(* FB_CylinderTempRecord	- number of control signals控制信号的数量:
									one direction is controllable一个方向是可控的
							- type of feedback signal反馈信号的类型:
									feedback in base and work position基准和工作位置的反馈
							- with temperature recording for data analysis具有用于数据分析的温度记录		*)

FUNCTION_BLOCK FB_CylinderTempRecord EXTENDS FB_CylinderTemp
VAR_INPUT
	bRecordStart		: BOOL;								// Signal to start the temperature recording开始温度记录的信号
	tIntervalTime		: TIME;								// Time of intervals to record the temperature记录温度的间隔时间 
END_VAR
VAR_OUTPUT
	bRecordDone			: BOOL;								// True if the temperature recording is done如果完成温度记录，则为True
	aTemps				: ARRAY[1..100] OF LREAL;			// Array with recorded temperatures用于记录温度的数组
END_VAR
VAR
	fbTimerInterval		: TON;								// Timer to control the recording interval控制记录间隔的计时器
	nIndex				: INT;								// Index to handle temperature array处理温度数组的索引
END_VAR

// =========================================================
;
// =========================================================

METHOD Record
VAR_INPUT
END_VAR
// =========================================================
// Recording array filled记录数组已填充
	
	bRecordDone := (nIndex = 100);

// =========================================================
// Recording temperatures记录温度
	
	IF bRecordStart AND NOT bRecordDone AND NOT fbTimerInterval.Q THEN
		fbTimerInterval(IN := TRUE,
						PT := tIntervalTime );
	END_IF
	
	IF fbTimerInterval.Q THEN
		fbTimerInterval(IN := FALSE);
		
		nIndex 			:= nIndex + 1;
		aTemps[nIndex] 	:= fTempCurrent;
	END_IF

// =========================================================
END_METHOD

METHOD Reset
VAR_INPUT
END_VAR
// =========================================================

// Calling method Reset of base class FB_Cylinder via 'SUPER^.'通过'SUPER^'调用FB_Cylinder的方法Reset
SUPER^.Reset();

// Reset temperature array重置温度数组
FOR nIndex := 1 TO 100 BY 1 DO
	aTemps[nIndex] := 0;
END_FOR

// Reset index重置索引
nIndex := 0;

// =========================================================
END_METHOD

END_FUNCTION_BLOCK
